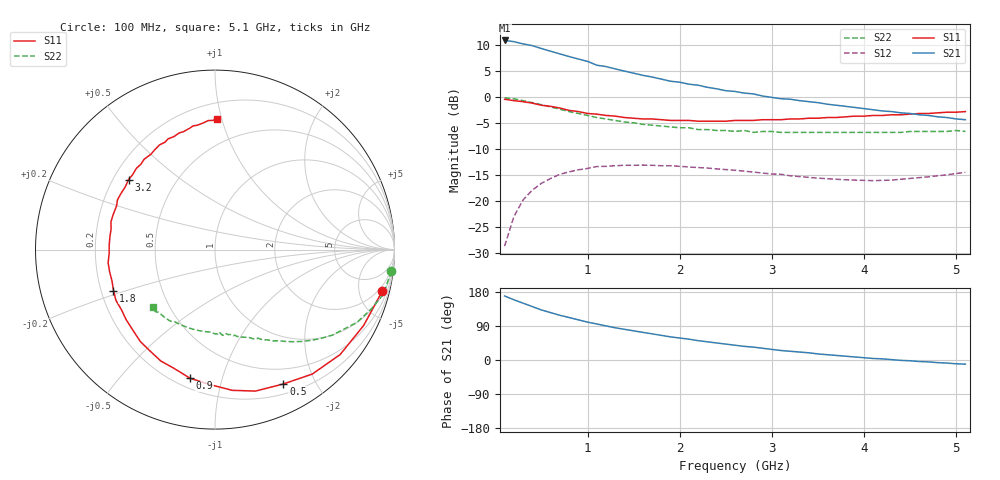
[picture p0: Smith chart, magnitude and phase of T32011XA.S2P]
!AT-32011
!S PARAMETERS at Vce=0.3 V  Ic=1mA.  LAST UPDATED 01-05-95
# ghz s ma r 50
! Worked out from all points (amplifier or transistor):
!   51 points, 100 MHz to 5.1 GHz, reference 50 ohm
!   highest |S21| = 11.0 dB at 100 MHz (marker M1)
!   |S21| within 3 dB of that: start of sweep to 780.2 MHz
!   unconditionally stable (mu >= 1): 2.496 GHz to end of sweep
!   at 900 MHz: K = 0.36, MSG = 10.7 dB, |S12| = -13.9 dB
!   at 2.6 GHz: K = 1.02, MAG = 6.7 dB, |S12| = -14.0 dB
!   at 5.1 GHz: K = 1.41, MAG = 1.2 dB, |S12| = -14.4 dB
!   S11 on the Smith chart (normalised r, x): 100 MHz: 1.34, -7.92; 500 MHz: 0.31, -1.59; 900 MHz: 0.26, -0.79; 1.8 GHz: 0.25, -0.18; 3.2 GHz: 0.26, +0.33; 5.1 GHz: 0.31, +0.97
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0.1  0.96 -14.0  3.53 169.0  0.037 83.0  0.99 -7.0
0.2  0.93 -27.0  3.44 159.0  0.071 72.0  0.97 -15.0
0.3  0.91 -40.0  3.27 150.0  0.103 64.0  0.93 -21.0
0.4  0.88 -52.0  3.15 141.0  0.128 57.0  0.89 -27.0
0.5  0.84 -63.0  2.95 132.0  0.149 51.0  0.85 -31.0
0.6  0.82 -74.0  2.78 125.0  0.166 45.0  0.81 -36.0
0.7  0.79 -83.0  2.62 118.0  0.182 40.0  0.77 -40.0
0.9  0.73 -101.0  2.34 106.0  0.201 31.0  0.7 -47.0
1  0.7 -109.0  2.22 100.0  0.207 28.0  0.67 -50.0
1.1  0.69 -116.0  2.04 95.0  0.216 23.0  0.64 -53.0
1.2  0.67 -123.0  1.98 90.0  0.217 21.0  0.62 -55.0
1.3  0.66 -129.0  1.88 85.0  0.22 18.0  0.6 -58.0
1.5  0.63 -142.0  1.71 77.0  0.222 13.0  0.57 -62.0
1.8  0.61 -158.0  1.5 65.0  0.22 7.0  0.53 -68.0
1.9  0.6 -163.0  1.43 61.0  0.22 5.0  0.52 -70.0
2.2  0.59 -178.0  1.31 51.0  0.211 0.0  0.49 -77.0
2.6  0.6 165.0  1.14 39.0  0.199 -4.0  0.47 -83.0
3.1  0.61 145.0  0.97 25.0  0.182 -6.0  0.46 -93.0
3.2  0.62 141.0  0.96 23.0  0.176 -5.0  0.46 -94.0
3.5  0.63 131.0  0.89 16.0  0.167 -4.0  0.46 -100.0
4.3  0.68 107.0  0.73 1.0  0.16 7.0  0.46 -117.0
5.1  0.73 89.0  0.61 -11.0  0.19 14.0  0.47 -137.0
